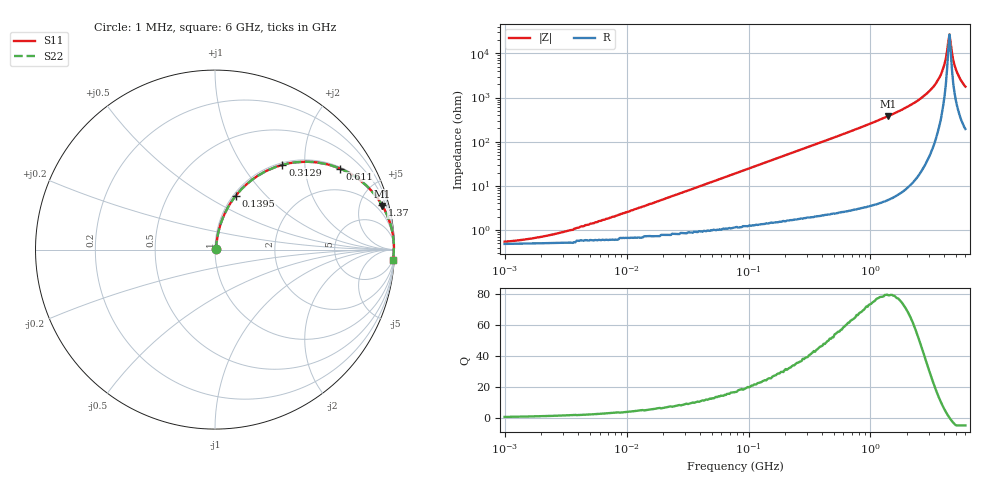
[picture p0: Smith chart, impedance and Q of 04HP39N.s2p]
# MHz S MA R 50
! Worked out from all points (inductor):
!   378 points, 1 MHz to 6 GHz, reference 50 ohm
!   read as one part in series: L = 39 nH near 7.445 MHz
!   highest Q = 79.2 at 1.402 GHz (marker M1), where L = 43.2 nH
!   self-resonance near 4.344 GHz
!   S11 on the Smith chart (normalised r, x): 1 MHz: 1.01, +0.00; 139.5 MHz: 1.03, +0.68; 312.9 MHz: 1.04, +1.54; 611 MHz: 1.05, +3.05; 1.37 GHz: 1.08, +7.43; 6 GHz: 5, -35
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1  0.005241 27.6  0.995 -0.1  0.995 -0.1  0.005241 27.6
2.093  0.007157 45.2  0.995 -0.3  0.995 -0.3  0.007157 45.2
4.279  0.012 61.4  0.994 -0.6  0.994 -0.6  0.012 61.4
18.312  0.045 78.0  0.992 -2.5  0.992 -2.5  0.045 78.0
78.359  0.187 75.8  0.971 -10.8  0.971 -10.8  0.187 75.8
139.517  0.32 69.0  0.934 -18.6  0.934 -18.6  0.32 69.0
312.884  0.603 51.5  0.783 -37.1  0.783 -37.1  0.603 51.5
335.312  0.63 49.6  0.762 -39.0  0.762 -39.0  0.63 49.6
610.957  0.83 32.9  0.544 -56.1  0.544 -56.1  0.83 32.9
1370.148  0.963 15.0  0.259 -74.2  0.259 -74.2  0.963 15.0
1402.133  0.964 14.6  0.253 -74.6  0.253 -74.6  0.964 14.6
1434.864  0.966 14.2  0.246 -75.0  0.246 -75.0  0.966 14.2
2383.891  0.991 6.9  0.121 -82.0  0.121 -82.0  0.991 6.9
3292.98  0.996 3.2  0.056 -84.2  0.056 -84.2  0.996 3.2
3695.704  0.997 1.9  0.034 -83.2  0.034 -83.2  0.997 1.9
3960.61  0.997 1.2  0.021 -80.3  0.021 -80.3  0.997 1.2
4147.681  0.997 0.7  0.013 -74.3  0.013 -74.3  0.997 0.7
4444.984  0.996 -0.0  0.003701 3.8  0.003701 3.8  0.996 -0.0
4654.933  0.996 -0.5  0.009551 64.9  0.009551 64.9  0.996 -0.5
4874.798  0.996 -1.0  0.018 75.0  0.018 75.0  0.996 -1.0
5470.975  0.994 -2.2  0.039 80.1  0.039 80.1  0.994 -2.2
6000  0.992 -3.2  0.056 80.5  0.056 80.5  0.992 -3.2
